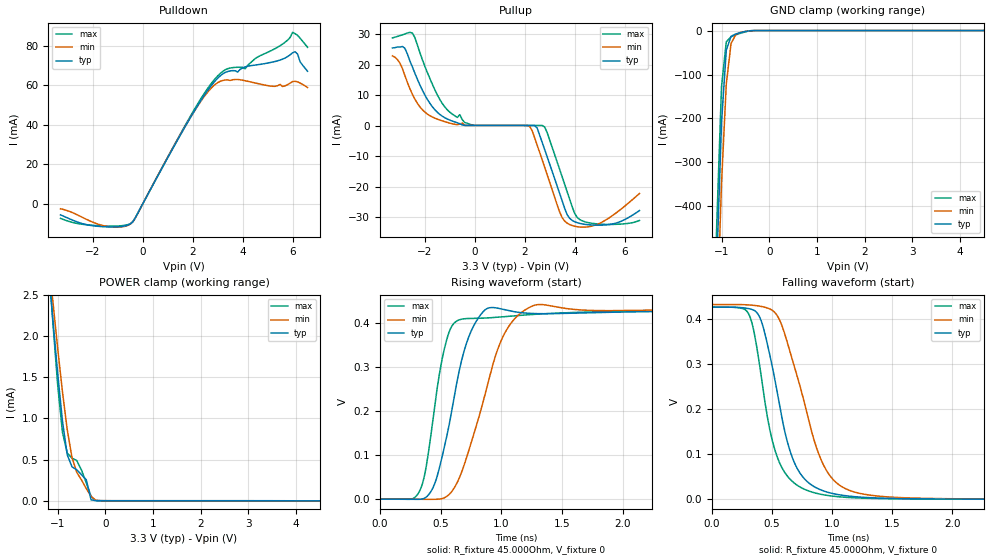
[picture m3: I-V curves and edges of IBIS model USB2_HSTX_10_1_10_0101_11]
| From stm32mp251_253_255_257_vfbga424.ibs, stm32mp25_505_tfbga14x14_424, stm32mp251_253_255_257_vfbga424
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[Model] USB2_HSTX_10_1_10_0101_11
Model_type   Output
Polarity   Non-Inverting
Enable   Active-High
C_comp   8.036pF   7.631pF   8.569pF
Vmeas = 200.000mV
Vref = 200.000mV
Rref = 45Ohms
Cref = 0pF
[Model Spec]
Vmeas   200.000mV   200.000mV   200.000mV
Vref   200.000mV   200.000mV   200.000mV
| This model is not intended for timing simulations.
| Warnings about Cref, Vref & Rref can be ignored
[Temperature Range]   25.000   125.000   -40.000
[Voltage Range]   3.300V   3.070V   3.630V
[GND Clamp Reference]   0.00V   0.00V   0.00V
[Pulldown Reference]   0.00V   0.00V   0.00V
[POWER Clamp Reference]   3.300V   3.070V   3.630V
[Pullup Reference]   3.300V   3.070V   3.630V
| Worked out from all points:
|   slope of the pulldown table from 0 to 0.495 V, typ, clamps not added: 42.6 ohm
|   GND clamp passes 1 mA (typ) near -0.43 V on its own axis
|   POWER clamp passes 1 mA (typ) near -0.91 V on its own axis
|   rising waveform, R_fixture 45.000Ohm, V_fixture 0: 20-80 % time 196ps typ, 274ps min, 143ps max; typ from 0 V to 0.428 V
|   falling waveform, R_fixture 45.000Ohm, V_fixture 0: 20-80 % time 216ps typ, 280ps min, 185ps max; typ from 0.427 V to 0 V
[GND Clamp]
-3.3V     -11.02A    -10.62A    -11.32A
-1.2V     -931.6mA   -1.049A    -855.7mA
-1.1V     -533.1mA   -671.7mA   -440.2mA
-1V       -209.4mA   -347mA     -127.3mA
-900mV    -44.44mA   -121.7mA   -25.59mA
-800mV    -13.15mA   -29.48mA   -14.15mA
-700mV    -7.742mA   -9.125mA   -9.769mA
-500mV    -2.127mA   -1.981mA   -2.894mA
-300mV    -19.29uA   -62.22uA   -13.53uA
6.6V      10.37uA    26.59uA    21.05uA
[Power Clamp]
-3.3V     3.206A     2.175A     4.855A
-1.2V     2.88mA     3.008mA    2.969mA
-1.1V     2.195mA    2.419mA    2.156mA
-1V       1.545mA    1.852mA    1.406mA
-900mV    967.9uA    1.324mA    831.4uA
-800mV    558.4uA    864.6uA    580.3uA
-700mV    412uA      525.9uA    517uA
-600mV    376.6uA    345uA      488.5uA
-400mV    254.2uA    146.6uA    216.8uA
-300mV    11.21uA    52.87uA    53.51uA
-100mV    94.94nA    984.9nA    361.1nA
6.6V      -3.577uA   -5.181uA   -3.995uA
[Pulldown]
-3.3V     -5.671mA   -2.581mA   -7.449mA
-1.6V     -11.64mA   -11.09mA   -11.31mA
-500mV    -10.25mA   -10.32mA   -10.1mA
1.9V      43.42mA    43.46mA    44.13mA
2.9V      62.15mA    60.37mA    63.26mA
3.4V      66.87mA    62.63mA    68.29mA
4.1V      69.19mA    62.19mA    68.26mA
4.5V      70.11mA    61.06mA    73.4mA
5.6V      73.12mA    59.29mA    80.76mA
6V        76.33mA    61.78mA    86.69mA
6.1V      76.87mA    61.92mA    85.99mA
6.6V      66.99mA    58.79mA    79.1mA
[Pullup]
-3.3V     25.41mA    22.83mA    28.67mA
-2.8V     25.3mA     16.37mA    30mA
-2.5V     19.22mA    10.28mA    30.28mA
-1.7V     6.185mA    2.827mA    13.54mA
-400mV    111.7uA    77.66uA    1.021mA
2.2V      68.59uA    -249uA     104.8uA
2.5V      -770.8uA   -6.355mA   83.46uA
2.8V      -7.785mA   -13.58mA   -409.6uA
3.4V      -22.12mA   -28.2mA    -14.26mA
3.8V      -30.28mA   -32.32mA   -24mA
4.4V      -32.24mA   -33.17mA   -31.39mA
6.6V      -27.75mA   -22.18mA   -30.98mA
[Ramp]
R_load=45.000Ohm
dV/dt_r   628.627mV/1.030ns  596.898mV/1.065ns  682.274mV/960.000ps
dV/dt_f   630.820mV/240.000ps  599.812mV/315.000ps  684.094mV/215.000ps
[Rising waveform]
R_fixture=45.000Ohm
V_fixture=0
0s        452.1nV    3.134uV    468nV
310ps     -466.1uV   -354.1uV   11.02mV
420ps     17.67mV    -467.7uV   147.4mV
500ps     83.02mV    475.1uV    301.7mV
580ps     184.3mV    13.74mV    386.9mV
720ps     360.4mV    100.4mV    410.3mV
910ps     435.1mV    286.2mV    412.1mV
1.07ns    427.7mV    396.3mV    415.6mV
1.31ns    421.4mV    442.2mV    420.5mV
9.9ns     427.9mV    433.7mV    427.8mV
[Falling waveform]
R_fixture=45.000Ohm
V_fixture=0
0s        427.4mV    433.2mV    427.3mV
310ps     423.7mV    432.1mV    409.5mV
410ps     396.3mV    428.9mV    273mV
540ps     241.5mV    409.4mV    95.91mV
620ps     134.7mV    354.7mV    54.04mV
700ps     73.11mV    281.9mV    32.94mV
950ps     16.68mV    65.04mV    9.054mV
1.17ns    6.32mV     17.4mV     3.525mV
1.69ns    1.195mV    2.668mV    853.9uV
9.9ns     14.12uV    30.97uV    4.491uV
